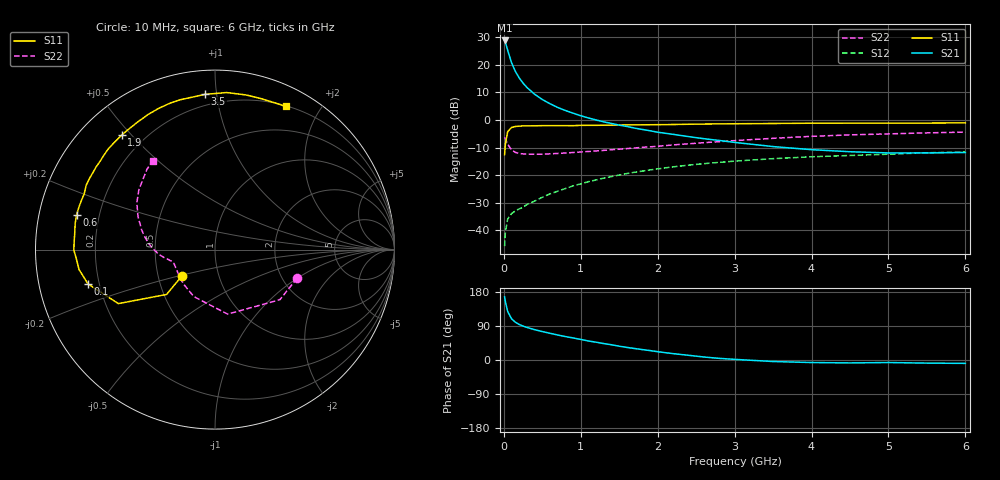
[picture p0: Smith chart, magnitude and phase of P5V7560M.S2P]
! SIEMENS Small Signal Semiconductors
! BFP183
! Si NPN RF Bipolar Junction Transistor in SOT143
! VCE = 0.75 V  IC = 60 mA
! Common Emitter S-Parameters:  March  1996
# GHz  S  MA  R  50
!  f  S11  S21  S12  S22
! GHz  MAG  ANG  MAG  ANG  MAG  ANG  MAG  ANG
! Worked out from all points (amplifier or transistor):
!   36 points, 10 MHz to 6 GHz, reference 50 ohm
!   highest |S21| = 28.8 dB at 10 MHz (marker M1)
!   |S21| within 3 dB of that: start of sweep to 44.17 MHz
!   unconditionally stable (mu >= 1): start of sweep to 41.27 MHz; 104.3 MHz to end of sweep
!   at 250 MHz: K = 1.56, MAG = 18.1 dB, |S12| = -31.6 dB
!   at 1.4 GHz: K = 2.11, MAG = 3.6 dB, |S12| = -20.4 dB
!   at 6 GHz: K = 1.51, MAG = -4.3 dB, |S12| = -11.6 dB
!   S11 on the Smith chart (normalised r, x): 10 MHz: 0.66, -0.21; 100 MHz: 0.16, -0.13; 600 MHz: 0.12, +0.12; 1.9 GHz: 0.12, +0.47; 3.5 GHz: 0.13, +0.93; 6 GHz: 0.21, +1.59
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0.01  0.2365 -141.5  27.67 166.4  0.0052 59.4  0.4846 -19.2
0.02  0.3677 -137.2  25.77 154.0  0.0093 58.4  0.4566 -37.7
0.05  0.6168 -150.8  18.34 127.9  0.0162 46.1  0.3663 -78.9
0.1  0.7332 -164.9  10.92 108.8  0.0202 36.9  0.2871 -114.3
0.15  0.7657 -171.7  7.61 99.6  0.0227 37.8  0.2599 -132.4
0.2  0.7746 -176.4  5.798 93.8  0.0246 41.7  0.2488 -142.2
0.25  0.7863 -179.8  4.669 89.4  0.0264 44.0  0.2435 -148.5
0.3  0.786 177.5  3.898 86.0  0.0295 47.5  0.2413 -152.9
0.4  0.787 173.1  2.941 80.0  0.0341 51.6  0.2408 -158.1
0.5  0.7927 169.4  2.355 75.1  0.04 54.2  0.2415 -161.1
0.6  0.7952 166.0  1.978 70.4  0.046 56.3  0.2446 -163.2
0.7  0.7943 162.7  1.694 66.0  0.0515 57.8  0.2486 -164.6
0.8  0.793 159.8  1.49 61.9  0.0575 58.3  0.2532 -165.7
1.1  0.8038 150.6  1.091 50.2  0.0766 58.1  0.27 -168.6
1.5  0.812 139.8  0.809 36.4  0.101 55.0  0.2968 -172.8
1.9  0.823 129.1  0.64 24.9  0.1249 50.3  0.3275 -178.0
2.2  0.8309 121.4  0.552 16.8  0.142 46.6  0.3549 177.5
2.8  0.8531 107.2  0.427 4.3  0.1714 38.4  0.4063 168.1
3.5  0.8668 93.6  0.331 -4.0  0.1998 29.4  0.4673 156.7
4.5  0.8788 78.6  0.267 -7.7  0.2282 17.2  0.5392 141.9
5.5  0.8825 68.1  0.254 -8.2  0.2556 7.3  0.5863 130.3
6  0.8903 63.7  0.259 -8.9  0.2643 2.0  0.6052 125.1
